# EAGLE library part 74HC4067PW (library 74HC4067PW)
1 Circuit IC Switch 16:1 120Ohm 24-TSSOP Source: Datasheet
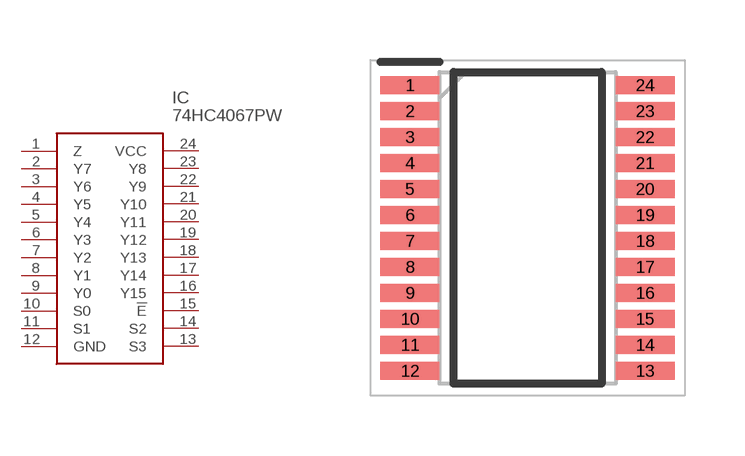
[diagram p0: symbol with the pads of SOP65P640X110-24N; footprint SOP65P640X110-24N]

Designator prefix IC

## 74HC4067PW (Description: 1 Circuit IC Switch 16:1 120Ohm 24-TSSOP; Height: 1.1mm; Manufacturer_Name: NXP; Manufacturer_Part_Number: 74HC4067PW)  [SOP65P640X110-24N]
1  Z
2  Y7
3  Y6
4  Y5
5  Y4
6  Y3
7  Y2
8  Y1
9  Y0
10  S0
11  S1
12  GND
13  S3
14  S2
15  !E
16  Y15
17  Y14
18  Y13
19  Y12
20  Y11
21  Y10
22  Y9
23  Y8
24  VCC

## Footprint SOP65P640X110-24N (pad centres in mm)
TSSOP24
smd 1.475 x 0.45: 1 -2.938,3.575; 2 -2.938,2.925; 3 -2.938,2.275; 4 -2.938,1.625; 5 -2.938,0.975; 6 -2.938,0.325; 7 -2.938,-0.325; 8 -2.938,-0.975; 9 -2.938,-1.625; 10 -2.938,-2.275; 11 -2.938,-2.925; 12 -2.938,-3.575; 13 2.938,-3.575; 14 2.938,-2.925; 15 2.938,-2.275; 16 2.938,-1.625; 17 2.938,-0.975; 18 2.938,-0.325; 19 2.938,0.325; 20 2.938,0.975; 21 2.938,1.625; 22 2.938,2.275; 23 2.938,2.925; 24 2.938,3.575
